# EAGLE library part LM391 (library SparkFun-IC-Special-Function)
LM3914 Dot/Bar Display Driver TTL/CMOS Logic Drives LEDs, LCDs, Vacuum Fluorecents Source: Data sheet LM3915 Data sheet LM3914 SparkFun Products: MyoWare LED Shield Dot/Bar Display Driver - LM3914
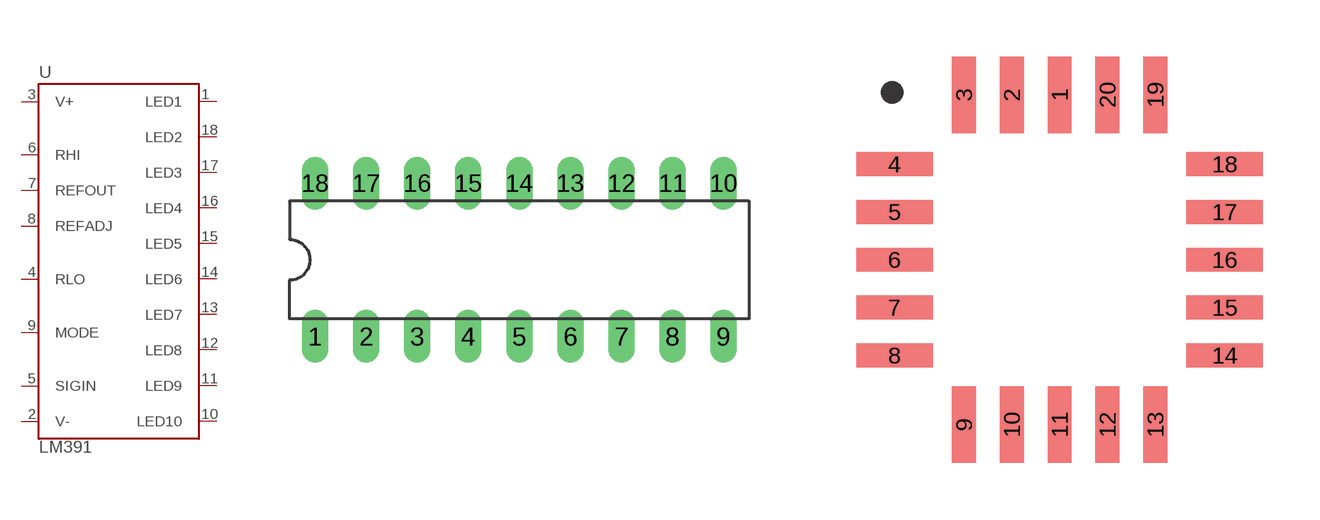
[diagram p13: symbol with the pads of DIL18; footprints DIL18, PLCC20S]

Designator prefix U

## LM391N (SF_ID: COM-12694), LM3914N, LM3915N  [DIL18]
1  LED1  out
2  V-  pwr
3  V+  pwr
4  RLO  in
5  SIGIN  in
6  RHI  in
7  REFOUT  out
8  REFADJ  pas
9  MODE  in
10  LED10  out
11  LED9  out
12  LED8  out
13  LED7  out
14  LED6  out
15  LED5  out
16  LED4  out
17  LED3  out
18  LED2  out

## LM391V, LM3914V (PROD_ID: IC-13110)  [PLCC20S]
1  LED1  out
2  V-  pwr
3  V+  pwr
4  RLO  in
5  SIGIN  in
6  RHI  in
8  REFOUT  out
10  REFADJ  pas
11  MODE  in
12  LED10  out
13  LED9  out
14  LED8  out
15  LED7  out
16  LED6  out
17  LED5  out
18  LED4  out
19  LED3  out
20  LED2  out

## Footprint DIL18 (pad centres in mm)
Dual In Line Package - 18 Pin Specifications: Pin count: 18 Example device(s): LM391
drill 0.813 long: 1 -10.16,-3.81; 2 -7.62,-3.81; 3 -5.08,-3.81; 4 -2.54,-3.81; 5 0,-3.81; 6 2.54,-3.81; 7 5.08,-3.81; 8 7.62,-3.81; 9 10.16,-3.81; 10 10.16,3.81; 11 7.62,3.81; 12 5.08,3.81; 13 2.54,3.81; 14 0,3.81; 15 -2.54,3.81; 16 -5.08,3.81; 17 -7.62,3.81; 18 -10.16,3.81

## Footprint PLCC20S (pad centres in mm)
PLCC 20 Pin Square Specifications: Pin count: 20 Datasheet referenced for footprint Example device(s): LM391
smd 0.63 x 2.035: 1 0,4.383; 2 -1.27,4.383; 3 -2.54,4.383; 9 -2.54,-4.383; 10 -1.27,-4.383; 11 0,-4.383; 12 1.27,-4.383; 13 2.54,-4.383; 19 2.54,4.383; 20 1.27,4.383
smd 2.035 x 0.63: 4 -4.383,2.54; 5 -4.383,1.27; 6 -4.383,0; 7 -4.383,-1.27; 8 -4.383,-2.54; 14 4.383,-2.54; 15 4.383,-1.27; 16 4.383,0; 17 4.383,1.27; 18 4.383,2.54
